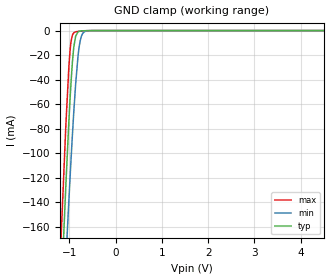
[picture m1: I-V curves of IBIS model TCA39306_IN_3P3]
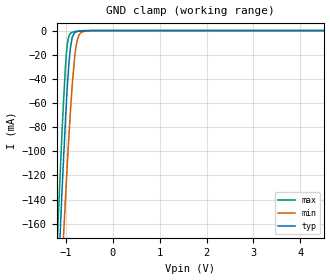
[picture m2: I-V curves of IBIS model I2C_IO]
|Texas Instruments Incorporated
| Low voltage FM+ I2C bus and SMBus voltage translator
| TCA39306
| Voltage Range : 0.9V-5.5V
| Package-type: DCU / DCT / DTM
| #pins/pkg drawing : 8-pin DCU /  8-pin DCT / 8-pin DTM
[IBIS Ver] 4.1
[File name] tca39306_3p3.ibs
[File Rev] 1.0
[Date] 07/01/2021
[Source]
| Texas Instruments Incorporated.
| 12500 TI Blvd
| Dallas, TX -75243
[Notes] Revision History:
| Rev 1.0: 07/01/2021
| - Initial version of the model
| - Model generated from simulations in SPECTRE
| - C_comp although listed in numerical order of value are
| obtained from varying PVT conditions. For PVT conditions for
| each specific value refer the buffer description under
| respective [Model]. IBIS model user is responsible for using
| appropriate C_comp to simulate for Signal Integrity.
| - Warnings regarding combined Non-monotonicity of various models have been
| reviewed and considered minor and can be ignored.
[Disclaimer]
| This model is designed as an aid for customers of Texas Instruments.
| TI and its licensors and suppliers make no warranties, either expressed
| or implied, with respect to this model, including the warranties of
| merchantability or fitness for a particular purpose. The model is
| provided solely on an "as is" basis. The entire risk as to its quality
| and performance is with the customer.
| This model is subject to change without notice. Texas Instruments
| Incorporated is not responsible for updating this model.
[Copyright]
(C) Copyright 2019 Texas Instruments Incorporated. All rights reserved.
| Component1 TCA39306DCU 8-PIN TSSOP
[Component] TCA39306_DCU
[Manufacturer] Texas Instruments Incorporated
[Package] |DCU 8-pin TSSOP
| variable typ   min   max
R_pkg 1.400e-02   1.300e-02   1.500e-02
L_pkg 1.289e-09   1.025e-09   2.014e-09
C_pkg 1.360e-13   6.600e-14   2.940e-13
[Pin]   signal_name   model_name   R_pin   L_pin   C_pin
1   GND   GND   1.400e-02   1.387e-09   1.760e-13
2   VREF1   I2C_IO   1.300e-02   1.026e-09   6.600e-14
3   SCL1   I2C_IO   1.300e-02   1.032e-09   6.700e-14
4   SDA1   I2C_IO   1.500e-02   2.014e-09   2.940e-13
5   SDA2   I2C_IO   1.400e-02   1.412e-09   1.780e-13
6   SCL2   I2C_IO   1.300e-02   1.030e-09   6.600e-14
7   VREF2   I2C_IO   1.300e-02   1.025e-09   6.600e-14
8   EN   TCA39306_IN   1.400e-02   1.386e-09   1.760e-13
[Series Pin Mapping]   pin_2   model_name   function_table_group
2   7   I2C_IO_S   1
3   6   I2C_IO_S   1
4   5   I2C_IO_S   1
[Series Switch Groups]
| Function Group States
On  1 /
Off 1 /
| Component2 TCA39306DCT 8-PIN TSSOP
[Component] TCA39306_DCT
[Manufacturer] Texas Instruments Incorporated
[Package] |DCU 8-pin TSSOP
| variable typ   min   max
R_pkg   2.900e-02   2.800e-02   3.100e-02
L_pkg   1.796e-09   1.666e-09   1.924e-09
C_pkg   1.090e-13   8.300e-14   1.360e-13
[Pin]   signal_name   model_name   R_pin   L_pin   C_pin
1   GND   GND   1.400e-02   1.387e-09   1.760e-13
2   VREF1   I2C_IO   1.300e-02   1.026e-09   6.600e-14
3   SCL1   I2C_IO   1.300e-02   1.032e-09   6.700e-14
4   SDA1   I2C_IO   1.500e-02   2.014e-09   2.940e-13
5   SDA2   I2C_IO   1.400e-02   1.412e-09   1.780e-13
6   SCL2   I2C_IO   1.300e-02   1.030e-09   6.600e-14
7   VREF2   I2C_IO   1.300e-02   1.025e-09   6.600e-14
8   EN   TCA39306_IN   1.400e-02   1.386e-09   1.760e-13
[Series Pin Mapping]   pin_2   model_name   function_table_group
2   7   I2C_IO_S   1
3   6   I2C_IO_S   1
4   5   I2C_IO_S   1
[Series Switch Groups]
| Function Group States
On 1 /
Off 1 /
| Component3 TCA39306DTM 8-PIN X2SON
[Component] TCA39306_DTM
[Manufacturer] Texas Instruments Incorporated
[Package] |DTM 8-pin X2SON
| variable typ   min   max
R_pkg   2.900e-02   2.800e-02   3.100e-02
L_pkg   1.796e-09   1.666e-09   1.924e-09
C_pkg   1.090e-13   8.300e-14   1.360e-13
[Pin]   signal_name   model_name   R_pin   L_pin   C_pin
1   GND   GND   3.000e-02   2.890e-10   7.058e-14
2   VREF1   I2C_IO   3.089e-02   2.672e-10   2.985e-13
3   SCL1   I2C_IO   3.203e-02   2.900e-10   .0654e-14
4   SDA1   I2C_IO   4.000e-02   4.124e-10   7.674e-13
5   SDA2   I2C_IO   3.190e-02   2.849e-10   1.780e-13
6   SCL2   I2C_IO   1.300e-02   2.664e-10   2.993e-13
7   VREF2   I2C_IO   3.206e-02   2.872e-10   6.541e-14
8   EN   TCA39306_IN   3.100e-02   2.839e-10   7.674e-13
[Series Pin Mapping]   pin_2   model_name   function_table_group
2   7   I2C_IO_S   1
3   6   I2C_IO_S   1
4   5   I2C_IO_S   1
[Series Switch Groups]
| Function Group States
On 1 /
Off 1 /
| I2C_IO_S
[Model]   I2C_IO_S
Model_type  Series_switch
| variable   typ   min   max
C_comp   2.6pF   2.2pF   3.5pF
[Temperature Range]   27   125   -40
[Voltage range]   3.3   3   3.6
[On]
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[Off]
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| Models and submodels in the file (3): TCA39306_IN_3P3 (Input), I2C_IO_S (Series_switch), I2C_IO (Terminator)
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| TCA39306_IN
[Model]   TCA39306_IN_3P3
Model_type   Input
Vinl=0.99
Vinh=2.31
|   typ   min   max
C_comp   11pF   9.4pF   13pF
[Voltage Range]   3.3   2.97   3.63
[Temperature Range]   27   125   -40
[Power Clamp Reference]   3.3   2.97   3.63
[GND Clamp Reference]   0   0   0
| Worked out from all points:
|   GND clamp passes 1 mA (typ) near -0.81 V on its own axis
[GND Clamp]
|   Voltage   I(typ)   I(min)   I(max)
-3.3V     -2.325A    -2.125A    -2.372A
-1.181V   -218.5mA   -271mA     -171.2mA
-1.171V   -209.5mA   -263mA     -161.9mA
-1.073V   -122.9mA   -184.7mA   -74.01mA
-1.013V   -75.52mA   -139.9mA   -30.85mA
-993.3mV  -61.12mA   -125.5mA   -20mA
-933.9mV  -25.17mA   -84.49mA   -3.541mA
-864.6mV  -4.514mA   -43.39mA   -1.013mA
-815.1mV  -1.138mA   -21.51mA   -696.5uA
-765.6mV  -411.5uA   -8.268mA   -494.6uA
-617.1mV  -53.19uA   -264.2uA   -109.9uA
6.6V      0A         0A         0A
| I2C_IO
[Model]   I2C_IO
Model_type   Terminator
|   typ   min   max
C_comp   2.6pF   2.2pF   3.5pF
[Voltage Range]   3.3   2.97   3.63
[Temperature Range]   27   125   -40
[Power Clamp Reference]   3.3   2.97   3.63
[GND Clamp Reference]   0   0   0
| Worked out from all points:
|   GND clamp passes 1 mA (typ) near -0.78 V on its own axis
[GND Clamp]
|   Voltage   I(typ)   I(min)   I(max)
-3.3V     -2.335A    -2.135A    -2.383A
-1.181V   -220.6mA   -273.5mA   -172.9mA
-1.171V   -211.6mA   -265.5mA   -163.6mA
-1.073V   -124.5mA   -186.9mA   -75.33mA
-1.013V   -76.98mA   -141.9mA   -31.95mA
-993.3mV  -62.52mA   -127.4mA   -21.03mA
-933.9mV  -26.38mA   -86.2mA    -4.306mA
-864.6mV  -5.457mA   -44.88mA   -1.369mA
-805.2mV  -1.532mA   -19.45mA   -750.1uA
-755.7mV  -737.5uA   -7.769mA   -476.1uA
-587.4mV  -39.63uA   -535.7uA   -69.65uA
6.6V      0A         0A         0A
